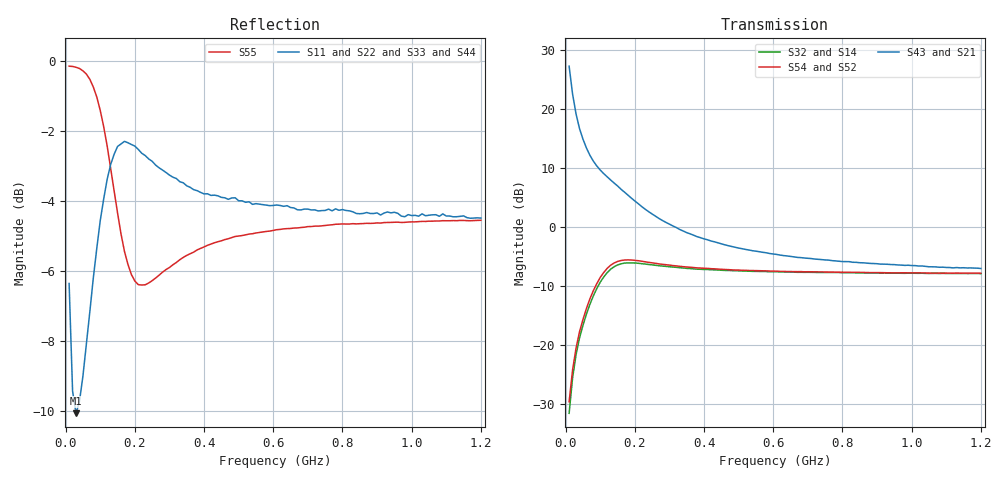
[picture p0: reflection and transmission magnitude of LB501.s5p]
!  POLYFET RF DEVICES
!  LB501 (Each Side)
!  S PARAMETERS
!  VDS=28V, IDQ=400mA
! Date: Thu Mar 13 09:54:24 2003
!AWR Design Environment (2053) Wed Feb 04 14:50:30 2004
!freq-unit  param-type  data-format  keyword  impedance-ohms
# MHz  S  MA  R  50
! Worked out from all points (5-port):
!   120 points, 10 MHz to 1.2 GHz, reference 50 ohm
!   strongest paths, dB at 10 MHz, 310 MHz, 610 MHz, 910 MHz, 1.2 GHz:
!     S43: 27.2, 0.2, -4.7, -6.3, -7.1
!     S21: 27.2, 0.2, -4.7, -6.3, -7.1
!     S54: -29.6, -6.6, -7.5, -7.8, -7.9
!     S52: -29.6, -6.6, -7.5, -7.8, -7.9
!     S32: -31.6, -6.8, -7.6, -7.8, -7.9
!     S14: -31.6, -6.8, -7.6, -7.8, -7.9
!   lowest |S11| = -10.1 dB at 30 MHz (marker M1), VSWR 1.91, Z = 52.7 - j33.8 ohm
!   |S11| at or under -10 dB: 28.77 MHz to 32.29 MHz (3.522 MHz wide, 11.5 % of centre)
